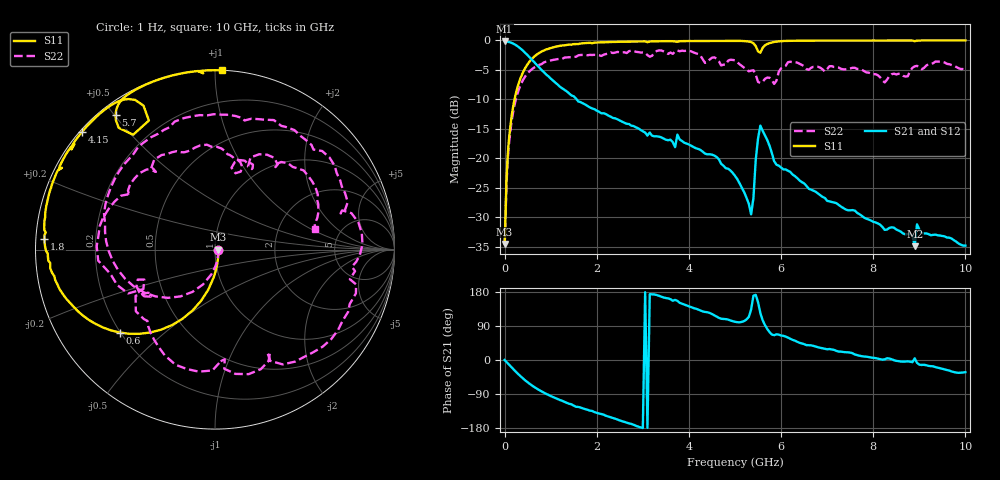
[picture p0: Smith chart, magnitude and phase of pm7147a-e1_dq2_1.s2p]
# GHz S DB R 50
! S-Parameters data
! Freq  dbS11  angS11  dbS21  angS21  dbS12  angS12  dbS22  angS22
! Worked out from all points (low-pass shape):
!   279 points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, 1 Hz to 10 GHz, reference 50 ohm
!   highest |S21| = -0.17 dB at 7.9 Hz (marker M1); lowest = -34.9 dB at 8.9 GHz (marker M2)
!   |S21| within 3 dB of the highest: start of sweep to 579.5 MHz
!   lowest |S11| = -34.5 dB at 15.8 Hz (marker M3), VSWR 1.04, Z = 51.9 - j1.96e-06 ohm
!   |S11| at or under -10 dB: start of sweep to 215.8 MHz
!   |S22| runs from -34.5 to -1.7 dB; largest |S21 - S12| = 0
!   S11 on the Smith chart (normalised r, x): 1 Hz: 1.04, -0.00; 600 MHz: 0.20, -0.36; 1.8 GHz: 0.02, +0.03; 4.15 GHz: 0.01, +0.38; 5.7 GHz: 0.04, +0.50; 10 GHz: 0.00, +1.04
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1e-09  -34.51 -0.0  -0.17 -0.0  -0.17 -0.0  -34.51 -0.0
7.9e-09  -34.51 -0.0  -0.17 -0.0  -0.17 -0.0  -34.51 -0.0
1.58e-08  -34.51 -0.0  -0.17 -0.0  -0.17 -0.0  -34.51 -0.0
0.06309573  -20.14 -84.8  -0.21 -8.2  -0.21 -8.2  -20.94 -87.9
0.15  -12.91 -99.5  -0.41 -19.4  -0.41 -19.4  -13.77 -108.9
0.6  -3.05 -138.9  -3.33 -67.8  -3.33 -67.8  -4.83 -173.8
1  -1.29 -160.1  -6.46 -95.1  -6.46 -95.1  -3.40 148.9
1.7  -0.47 178.9  -10.67 -127.7  -10.67 -127.7  -2.46 99.8
1.8  -0.43 176.5  -11.12 -131.4  -11.12 -131.4  -2.51 93.4
2.45  -0.24 163.6  -13.38 -157.4  -13.38 -157.4  -1.94 56.4
3.35  -0.14 149.4  -16.32 169.4  -16.32 169.4  -1.69 6.4
4.15  -0.09 138.5  -18.28 135.3  -18.28 135.3  -2.18 -50.1
5.05  -0.07 126.4  -23.52 99.8  -23.52 99.8  -3.72 -115.5
5.35  -0.27 120.0  -29.49 133.3  -29.49 133.3  -5.13 -135.7
5.55  -2.09 125.5  -14.45 124.0  -14.45 124.0  -7.21 -146.2
5.7  -0.61 126.4  -16.90 82.0  -16.90 82.0  -6.30 -150.5
6.2  -0.07 118.5  -22.29 55.9  -22.29 55.9  -3.62 178.3
6.7  -0.03 113.1  -25.48 37.3  -25.48 37.3  -4.48 142.2
8.35  -0.01 98.9  -31.79 3.9  -31.79 3.9  -6.03 77.3
8.9  -0.14 93.8  -34.89 4.3  -34.89 4.3  -4.39 61.2
8.95  -0.03 95.2  -31.19 -7.6  -31.19 -7.6  -4.31 57.0
10  -0.00 87.7  -34.80 -32.1  -34.80 -32.1  -4.90 11.4
